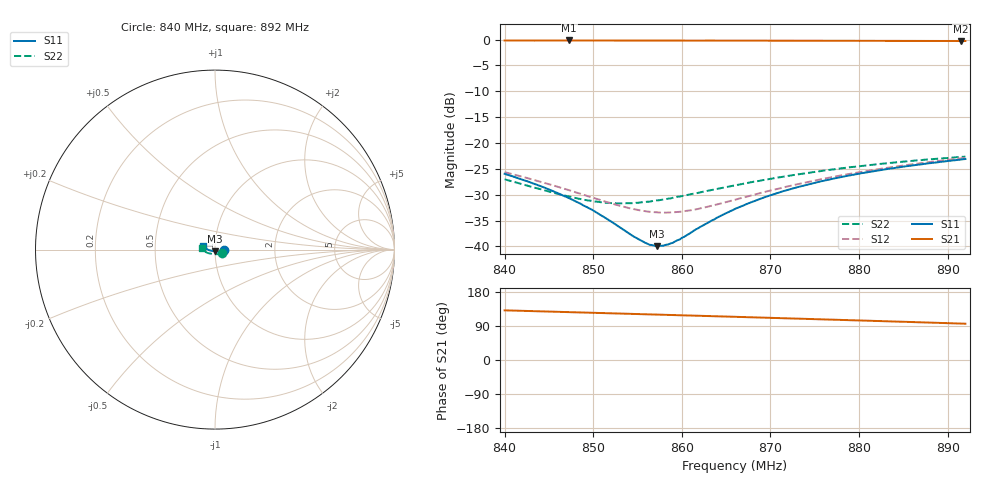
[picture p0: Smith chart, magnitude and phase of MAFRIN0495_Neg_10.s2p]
!Part Number:  MAFRIN0495
!Name:  MariaCraven
!Comments:  1
!Thu 30/Sep/2004  3:29:06 PM
!Temperature:  -10
# MHZ  S  DB  R  50
!Freq  S11(dB)  S11(ang)  S21(dB)  S21(ang)  S12(dB)  S12(ang)  S22(dB)  S22(ang)
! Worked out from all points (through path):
!   201 points, 840 MHz to 892 MHz, reference 50 ohm
!   highest |S21| = -0.18 dB at 847.3 MHz (marker M1); lowest = -0.3 dB at 891.5 MHz (marker M2)
!   group delay of S21, straight-line fit = 1.88 ns
!   lowest |S11| = -39.9 dB at 857.2 MHz (marker M3), VSWR 1.02, Z = 49.8 - j0.984 ohm
!   |S11| at or under -10 dB: start of sweep to end of sweep
!   |S22| runs from -31.7 to -22.6 dB; largest |S21 - S12| = 1
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840  -25.96 -4.9  -0.20 131.0  -25.64 105.7  -27.00 -27.8
844.42  -28.57 -12.0  -0.19 128.2  -27.67 109.9  -29.12 -43.7
847.28  -30.67 -18.5  -0.18 126.3  -29.12 115.0  -30.35 -57.5
848.84  -32.03 -23.7  -0.19 125.3  -29.98 119.0  -30.93 -66.0
849.88  -32.92 -27.3  -0.19 124.6  -30.54 122.2  -31.20 -71.9
852.74  -36.01 -44.9  -0.19 122.8  -32.01 133.7  -31.67 -89.5
854.56  -38.07 -63.1  -0.20 121.5  -32.76 143.1  -31.63 -100.6
855.86  -39.28 -81.7  -0.20 120.7  -33.17 150.7  -31.38 -107.9
856.38  -39.69 -89.3  -0.20 120.4  -33.30 153.8  -31.34 -110.6
857.16  -39.94 -101.0  -0.19 119.9  -33.39 158.6  -31.09 -114.5
857.42  -39.86 -104.8  -0.20 119.7  -33.44 160.3  -31.06 -115.6
857.94  -39.83 -112.1  -0.19 119.3  -33.46 163.3  -30.92 -118.2
858.98  -39.30 -124.7  -0.20 118.6  -33.40 169.5  -30.59 -122.9
861.84  -36.48 -148.2  -0.21 116.7  -32.75 -176.3  -29.63 -134.1
866  -32.73 -164.4  -0.22 113.9  -30.97 -162.4  -28.20 -146.7
869.38  -30.46 -171.9  -0.22 111.7  -29.45 -156.1  -27.12 -154.4
871.46  -29.30 -175.3  -0.23 110.3  -28.58 -153.4  -26.52 -158.3
874.84  -27.76 179.7  -0.24 107.9  -27.32 -150.8  -25.63 -164.3
878.74  -26.33 175.0  -0.24 105.2  -26.03 -149.3  -24.75 -170.1
883.42  -24.97 170.1  -0.27 101.9  -24.73 -148.8  -23.86 -176.6
891.48  -23.20 162.1  -0.29 96.1  -22.98 -149.7  -22.70 173.5
892  -23.09 161.6  -0.29 95.8  -22.87 -149.9  -22.64 173.0
